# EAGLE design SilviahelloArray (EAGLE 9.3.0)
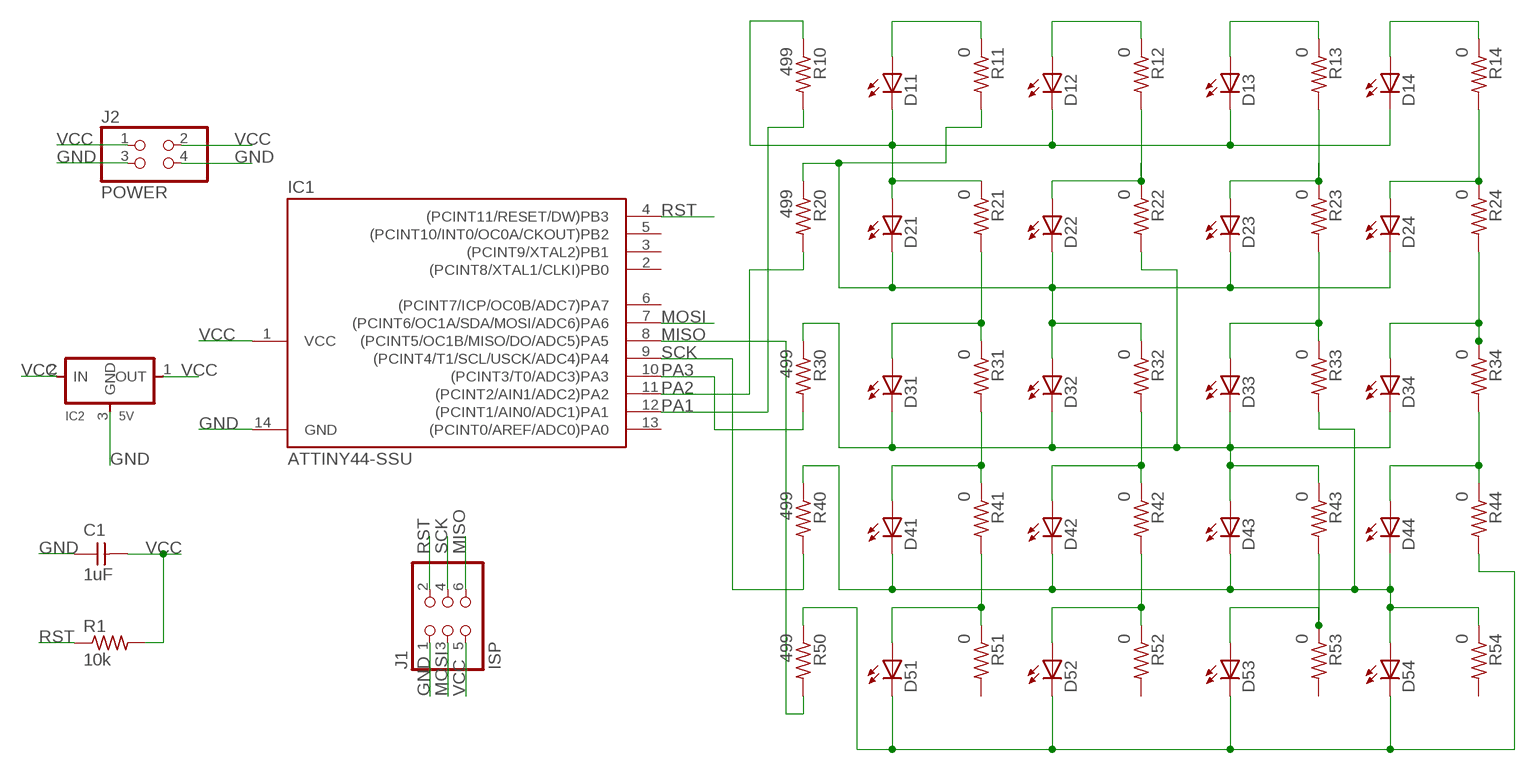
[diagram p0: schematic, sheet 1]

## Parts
C1  1uF  UNPOLARIZED_CAPACITOR1206  [1206]
D11  LED1206  [1206]
D12  LED1206  [1206]
D13  LED1206  [1206]
D14  LED1206  [1206]
D21  LED1206  [1206]
D22  LED1206  [1206]
D23  LED1206  [1206]
D24  LED1206  [1206]
D31  LED1206  [1206]
D32  LED1206  [1206]
D33  LED1206  [1206]
D34  LED1206  [1206]
D41  LED1206  [1206]
D42  LED1206  [1206]
D43  LED1206  [1206]
D44  LED1206  [1206]
D51  LED1206  [1206]
D52  LED1206  [1206]
D53  LED1206  [1206]
D54  LED1206  [1206]
IC1  ATTINY44-SSU  [SOIC14]
IC2  5V  REGULATORSOT23  [SOT23]
J1  ISP  PINHD-2X3-SMD  [2X03SMD]
J2  POWER  PINHD-2X2-SMD  [2X02SMD]
R1  10k  RESISTOR1206  [1206]
R10  499  RESISTOR1206  [1206]
R11  0  RESISTOR1206  [1206]
R12  0  RESISTOR1206  [1206]
R13  0  RESISTOR1206  [1206]
R14  0  RESISTOR1206  [1206]
R20  499  RESISTOR1206  [1206]
R21  0  RESISTOR1206  [1206]
R22  0  RESISTOR1206  [1206]
R23  0  RESISTOR1206  [1206]
R24  0  RESISTOR1206  [1206]
R30  499  RESISTOR1206  [1206]
R31  0  RESISTOR1206  [1206]
R32  0  RESISTOR1206  [1206]
R33  0  RESISTOR1206  [1206]
R34  0  RESISTOR1206  [1206]
R40  499  RESISTOR1206  [1206]
R41  0  RESISTOR1206  [1206]
R42  0  RESISTOR1206  [1206]
R43  0  RESISTOR1206  [1206]
R44  0  RESISTOR1206  [1206]
R50  499  RESISTOR1206  [1206]
R51  0  RESISTOR1206  [1206]
R52  0  RESISTOR1206  [1206]
R53  0  RESISTOR1206  [1206]
R54  0  RESISTOR1206  [1206]

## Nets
GND: C1.1 IC1.14(GND) IC2.3(GND) J1.1 J2.3 J2.4
MISO: IC1.8((PCINT5/OC1B/MISO/DO/ADC5)PA5) J1.6 R50.2
MOSI: IC1.7((PCINT6/OC1A/SDA/MOSI/ADC6)PA6) J1.3
N$34: D11.1(A) R11.1
N$53: D21.2(C) D22.2(C) D23.2(C) D24.2(C) D32.1(A) R11.2 R20.1 R32.1
N$55: D31.1(A) R21.2 R31.1
N$57: D41.1(A) R31.2 R41.1
N$59: D51.1(A) R41.2 R51.1
N$62: D12.1(A) R12.1
N$73: D22.1(A) R12.2 R22.1
N$75: D31.2(C) D32.2(C) D33.2(C) D34.2(C) D43.1(A) R22.2 R30.1 R43.1
N$77: D42.1(A) R32.2 R42.1
N$79: D52.1(A) R42.2 R52.1
N$82: D13.1(A) R13.1
N$83: D11.2(C) D12.2(C) D13.2(C) D14.2(C) D21.1(A) R10.1 R21.1
N$89: D41.2(C) D42.2(C) D43.2(C) D44.2(C) D54.1(A) R33.2 R40.1 R54.1
N$93: D23.1(A) R13.2 R23.1
N$95: D33.1(A) R23.2 R33.1
N$99: D53.1(A) R43.2 R53.1
N$102: D14.1(A) R14.1
N$104: D24.1(A) R14.2 R24.1
N$106: D34.1(A) R24.2 R34.1
N$108: D44.1(A) R34.2 R44.1
N$111: D51.2(C) D52.2(C) D53.2(C) D54.2(C) R44.2 R50.1
PA1: IC1.12((PCINT1/AIN0/ADC1)PA1) R10.2
PA2: IC1.11((PCINT2/AIN1/ADC2)PA2) R20.2
PA3: IC1.10((PCINT3/T0/ADC3)PA3) R30.2
RST: IC1.4((PCINT11/RESET/DW)PB3) J1.2 R1.1
SCK: IC1.9((PCINT4/T1/SCL/USCK/ADC4)PA4) J1.4 R40.2
VCC: C1.2 IC1.1(VCC) IC2.1(OUT) IC2.2(IN) J1.5 J2.1 J2.2 R1.2
Unconnected: IC1.2((PCINT8/XTAL1/CLKI)PB0) IC1.3((PCINT9/XTAL2)PB1) IC1.5((PCINT10/INT0/OC0A/CKOUT)PB2) IC1.6((PCINT7/ICP/OC0B/ADC7)PA7) IC1.13((PCINT0/AREF/ADC0)PA0) R51.2 R52.2 R53.2 R54.2

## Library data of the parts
C1 = 01_ng:UNPOLARIZED_CAPACITOR: unpolarized_capacitor
D11-D14 D21-D24 D31-D34 D41-D44 D51-D54 = 01_ng:LED
IC1 = 01_FAB_Hello:ATTINY44
IC2 = 01_ng:REGULATOR
J1 = 01_fab:PINHD-2X3-SMD: PIN HEADER
J2 = 01_fab:PINHD-2X2-SMD
R1 R10-R14 R20-R24 R30-R34 R40-R44 R50-R54 = 01_ng:RESISTOR

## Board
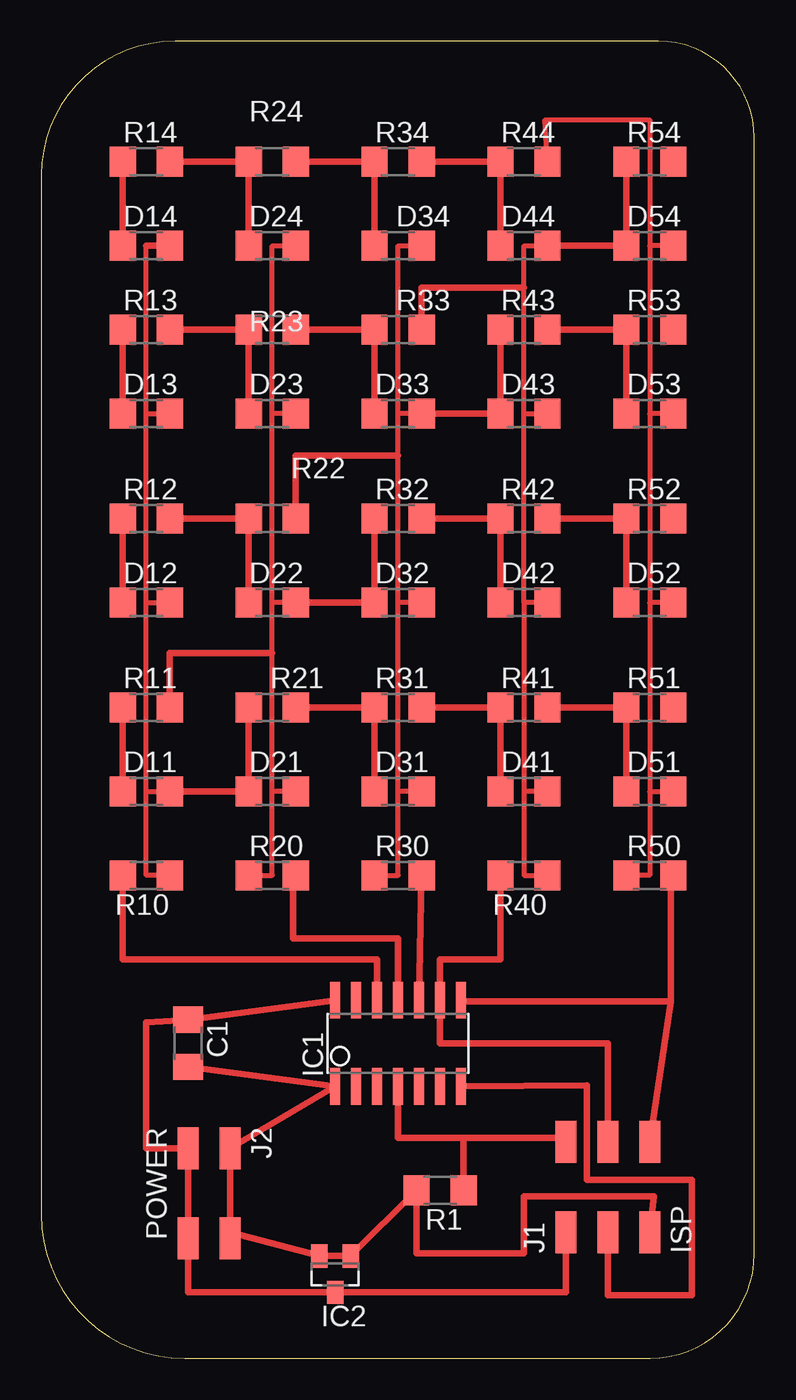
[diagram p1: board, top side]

Size 43.16 x 79.68 mm. Coordinates in mm from the lower left corner, seen from the top.
Outline: 0,71.58 0,8.67 arc90 8.67,0 36.85,0 arc90 43.16,6.31 43.16,73.87 arc90 37.35,79.68 8.1,79.68 arc90 0,71.58
Copper layers (1*16): Top 0.035mm / dielectric 1.5mm / Bottom 0.035mm
Design rules "default": minimum track width 6mil, minimum drill 0.35mm, track to track 6mil, track to pad 6mil, pad to pad 6mil, via to via 6mil, smd to smd 6mil, copper to edge 40mil, drill to drill 6mil, minimum pad ring 10mil, minimum via ring 8mil, stop-mask expansion 4mil, vias tented up to drill 0mil, thermal gap 10mil

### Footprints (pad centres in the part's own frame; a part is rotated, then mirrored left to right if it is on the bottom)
1206 = smd 1.6 x 1.803: 1 -1.422,0; 2 1.422,0
SOIC14 = smd 0.61 x 2.21: 1 -3.81,-2.603; 2 -2.54,-2.603; 3 -1.27,-2.603; 4 0,-2.603; 5 1.27,-2.603; 6 2.54,-2.603; 7 3.81,-2.603; 8 3.81,2.603; 9 2.54,2.603; 10 1.27,2.603; 11 0,2.603; 12 -1.27,2.603; 13 -2.54,2.603; 14 -3.81,2.603
SOT23 = smd 1 x 1.4: 1 -0.95,-1.1; 2 0.95,-1.1; 3 0,1.1
2X03SMD = smd 2.54 x 1.27: 1 -2.54,2.54; 2 2.92,2.54; 3 -2.54,0; 4 2.92,0; 5 -2.54,-2.54; 6 2.92,-2.54
2X02SMD = smd 2.54 x 1.27: 1 -2.54,1.27; 2 2.92,1.27; 3 -2.54,-1.27; 4 2.92,-1.27

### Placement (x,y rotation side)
C1  8.89,19.05 270 top
D11  6.35,34.29 0 top
D12  6.35,45.72 0 top
D13  6.35,57.15 0 top
D14  6.35,67.31 0 top
D21  13.97,34.29 0 top
D22  13.97,45.72 0 top
D23  13.97,57.15 0 top
D24  13.97,67.31 0 top
D31  21.59,34.29 0 top
D32  21.59,45.72 0 top
D33  21.59,57.15 0 top
D34  21.59,67.31 0 top
D41  29.21,34.29 0 top
D42  29.21,45.72 0 top
D43  29.21,57.15 0 top
D44  29.21,67.31 0 top
D51  36.83,34.29 0 top
D52  36.83,45.72 0 top
D53  36.83,57.15 0 top
D54  36.83,67.31 0 top
IC1  21.59,19.05 0 top
IC2  17.78,5.08 180 top
J1  34.29,10.16 90 top
J2  10.16,10.16 270 top
R1  24.13,10.16 180 top
R10  6.35,29.21 180 top
R11  6.35,39.37 0 top
R12  6.35,50.8 0 top
R13  6.35,62.23 0 top
R14  6.35,72.39 0 top
R20  13.97,29.21 0 top
R21  13.97,39.37 0 top
R22  13.97,50.8 0 top
R23  13.97,62.23 0 top
R24  13.97,72.39 0 top
R30  21.59,29.21 0 top
R31  21.59,39.37 0 top
R32  21.59,50.8 0 top
R33  21.59,62.23 0 top
R34  21.59,72.39 0 top
R40  29.21,29.21 180 top
R41  29.21,39.37 0 top
R42  29.21,50.8 0 top
R43  29.21,62.23 0 top
R44  29.21,72.39 0 top
R50  36.83,29.21 0 top
R51  36.83,39.37 0 top
R52  36.83,50.8 0 top
R53  36.83,62.23 0 top
R54  36.83,72.39 0 top

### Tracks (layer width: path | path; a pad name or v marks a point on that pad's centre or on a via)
GND
  Top 0.406: J1.1 31.75,3.98 IC2.3 8.89,3.98 J2.4 J2.3 6.35,12.7 6.35,20.32 C1.1 IC1.14
MISO
  Top 0.152: J1.6 36.42,13.49 | IC1.8 25.4,21.59 | 38.1,29.21 R50.2
  Top 0.406: 25.4,21.59 38.1,21.59 | 38.1,21.59 38.1,29.21 | 38.1,21.59 J1.6
MOSI
  Top 0.406: J1.3 34.29,3.81 39.37,3.81 39.37,10.79 33.02,10.79 33.02,16.51 IC1.7
N$34
  Top 0.406: D11.1 R11.1
N$53
  Top 0.152: 15.24,57.15 D23.2 | R32.1 20.32,50.8
  Top 0.305: R20.1 13.97,29.21 13.97,34.29 | 13.97,34.29 13.97,42.67 13.97,45.72 | 13.97,45.72 13.97,57.15 | 13.97,57.15 13.97,67.31 D24.2 | D21.2 13.97,34.29 | D22.2 13.97,45.72 | D23.2 13.97,57.15
  Top 0.406: R11.2 7.77,42.67 13.97,42.67 | R32.1 D32.1 D22.2
N$55
  Top 0.406: D31.1 R31.1 R21.2
N$57
  Top 0.406: R31.2 R41.1 D41.1
N$59
  Top 0.406: D51.1 R51.1 R41.2
N$62
  Top 0.406: D12.1 R12.1
N$73
  Top 0.406: D22.1 R22.1 R12.2
N$75
  Top 0.152: R22.2 15.24,50.8
  Top 0.305: R30.1 21.59,29.21 21.59,34.29 | 21.59,34.29 21.59,45.72 | 21.59,45.72 21.59,54.61 21.59,57.15 | 21.59,57.15 21.59,67.31 D34.2 | D31.2 21.59,34.29 | D33.2 21.59,57.15 | D32.2 21.59,45.72
  Top 0.406: D33.2 D43.1 R43.1 | R22.2 15.39,54.61 21.59,54.61
N$77
  Top 0.406: R32.2 R42.1 D42.1
N$79
  Top 0.406: D52.1 R52.1 R42.2
N$82
  Top 0.406: D13.1 R13.1
N$83
  Top 0.152: 7.62,34.29 D11.2
  Top 0.305: R10.1 6.35,29.21 6.35,34.29 | 6.35,34.29 6.35,45.72 | 6.35,45.72 6.35,57.15 | 6.35,57.15 6.35,67.31 | 6.35,57.15 D13.2 | 6.35,45.72 D12.2 | 6.35,34.29 7.62,34.29
  Top 0.406: R21.1 D21.1 D11.2 | 6.35,67.31 D14.2
N$89
  Top 0.152: 22.86,62.23 R33.2
  Top 0.305: D41.2 29.21,34.29 | 29.21,45.72 29.21,34.29 | D42.2 29.21,45.72 | 29.21,45.72 29.21,57.15 | 29.21,57.15 D43.2 | 29.21,34.29 29.21,29.21 R40.1 | D44.2 29.21,67.31 29.21,64.77 29.21,57.15
  Top 0.406: R54.1 D54.1 D44.2 | R33.2 23.01,64.77 29.21,64.77
N$93
  Top 0.406: D23.1 R23.1 R13.2
N$95
  Top 0.406: R23.2 R33.1 D33.1
N$99
  Top 0.406: D53.1 R53.1 R43.2
N$102
  Top 0.406: D14.1 R14.1
N$104
  Top 0.406: R14.2 R24.1 D24.1
N$106
  Top 0.406: R24.2 R34.1 D34.1
N$108
  Top 0.406: R34.2 R44.1 D44.1
N$111
  Top 0.305: R44.2 30.48,74.93 36.83,74.93 36.83,67.31 | 36.83,67.31 36.83,57.15 | 36.83,57.15 36.83,45.72 | 36.83,45.72 36.83,34.29 | 36.83,34.29 36.83,29.21 R50.1 | 36.83,34.29 D51.2 | D52.2 36.83,45.72 | D54.2 36.83,67.31 | D53.2 36.83,57.15
PA1
  Top 0.254: 5.08,24.13 4.93,24.13
  Top 0.406: IC1.12 20.32,24.13 5.08,24.13 | 4.93,24.13 R10.2
PA2
  Top 0.152: 15.24,29.21 R20.2
  Top 0.406: IC1.11 21.59,25.4 15.24,25.4 15.24,29.21
PA3
  Top 0.406: IC1.10 R30.2
RST
  Top 0.152: R1.1 25.4,10.31 | 31.37,12.7 J1.2 31.49,13.33 | 25.55,13.18 25.4,13.33
  Top 0.406: IC1.4 21.59,13.33 25.4,13.33 31.49,13.33 | R1.1 25.55,13.18
SCK
  Top 0.406: J1.4 34.29,19.05 24.13,19.05 IC1.9 24.13,24.13 27.79,24.13 R40.2
VCC
  Top 0.152: 18.9,6.35 arc90 IC2.1 | J2.2 11.43,7.62
  Top 0.406: IC2.1 R1.2 22.71,6.35 29.21,6.35 29.21,9.78 37.08,9.78 J1.5 | IC2.1 IC2.2 11.43,7.62 J2.1 IC1.1 C1.2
